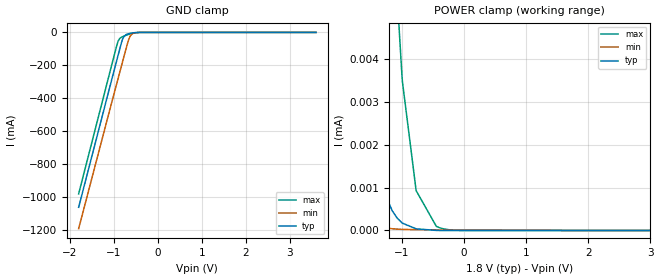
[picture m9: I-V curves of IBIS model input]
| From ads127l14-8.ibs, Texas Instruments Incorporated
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|   input Model
[Model]   input
Model_type   Input
Vinl = 0.54
Vinh = 1.26
|   typ   min   max
C_comp   0.382pF   0.386pF   0.377pF
[Voltage Range]   1.8   1.65   1.95
[Temperature Range]   27   125   -40
[Power Clamp Reference]   1.8   1.65   1.95
[GND Clamp Reference]   0   0   0
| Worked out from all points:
|   GND clamp passes 1 mA (typ) near -0.48 V on its own axis
[GND Clamp]
|   Voltage   I(typ)   I(min)   I(max)
-1.8V     -1.065A    -1.195A    -982.9mA
-1.066V   -306mA     -445mA     -216.7mA
-909mV    -145.9mA   -287.4mA   -58.43mA
-865.8mV  -102.2mA   -243.9mA   -37.06mA
-811.8mV  -49.84mA   -189.7mA   -27.37mA
-768.6mV  -24.81mA   -146.5mA   -22.54mA
-666mV    -8.238mA   -47.02mA   -12.3mA
-628.2mV  -5.842mA   -23.5mA    -9.055mA
-590.4mV  -3.95mA    -10.62mA   -6.243mA
-536.4mV  -1.988mA   -3.295mA   -3.17mA
-379.8mV  -73.29uA   -116.7uA   -105.6uA
3.6V      0A         0A         0A
[POWER Clamp]
|   Voltage   I(typ)   I(min)   I(max)
-1.8V     11.43uA    829.3nA    114.9uA
-1.611V   4.958uA    329nA      61.11uA
-1.579V   4.262uA    280nA      54.18uA
-1.503V   2.967uA    192nA      40.47uA
-1.444V   2.21uA     143.1nA    31.67uA
-1.379V   1.588uA    104.6nA    24.1uA
-1.233V   724.7nA    54.6nA     12.25uA
-1.071V   282.7nA    31.24nA    5.411uA
-990mV    171.2nA    25.64nA    3.482uA
-768.6mV  38.07nA    18.71nA    929.5nA
-444.6mV  1.62nA     15.26nA    98.29nA
3.6V      0A         0A         0A
